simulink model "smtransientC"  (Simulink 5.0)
settings: Solver=ode45  StartTime=0.0  StopTime=2  MaxStep=1e-3  RelTol=1e-4  AbsTol=1e-4
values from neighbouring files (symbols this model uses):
  Bm = 0.10    (= 0.1)    [IMabc2.m]    (also in imabcparam.m = 0.01; IMabcrun0.m = 0.01; IMabcrun1.m = 0.001; IMcur0.m = 1e-06)
  H = 0.60    (= 0.6)    [IMabc2.m]    (also in IMcur0.m = 0.3; imdef0vec.m = 0.3; imdef1vec.m = 0.3; imdef2vec.m = 0.3)
  n0 = 0.98    [imdef0vec.m]    (also in imdef1vec.m = 0.978; imdef2vec.m; imdefrotflux.m; imdefSIvec1.m = 0.95)
  tc = abs(fco)    [im3phase.m]
  Te0 = 0.75/wo*p*(Is*conj(Is)*Req)    [imdefSIvec1.m]
  V = [Vas 0 0].'    [Actac.m]    (also in acttrcalc1.m = str2num(get(h,'string')); im3d.m = eval(get(hVs,'String')); IMabc2.m = [vas vbs vcs 0 0 0]'; IMabcf0.m = [vas vbs vcs 0 0 0]')
  wo = 2*pi*freq0    [calc0.m]    (also in IMabc2.m = 376.991118431; imabcparam.m = 376.991118431; IMabcrun0.m = 376.991118431; IMabcrun1.m = 376.991118431)
undefined symbols (not defined in the file or in its folder): delta0, Lw_1, phif0
libraries: simulink x1

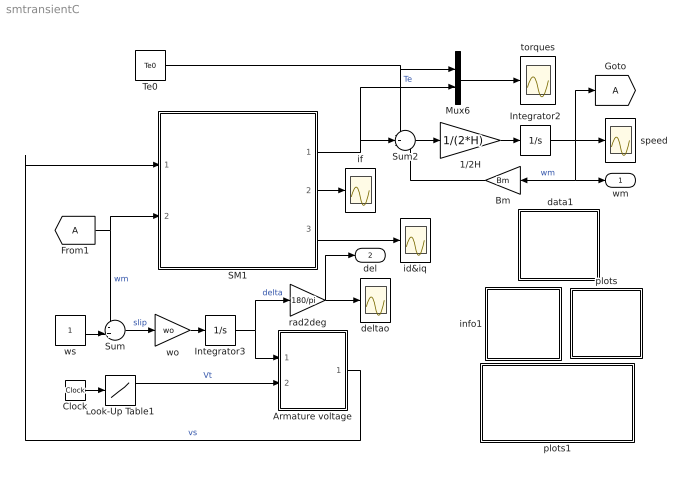
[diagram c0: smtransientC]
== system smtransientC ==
  " data1" : Subsystem
  1/2H : Gain  Gain=1/(2*H)
  Armature voltage : Subsystem
  Bm : Gain  Orientation=left  Gain=Bm
  Clock : Clock
  Integrator2 : Integrator  InitialCondition=n0
  Integrator3 : Integrator  InitialCondition=delta0
  Look-Up Table1 : Lookup  InputValues=[0 0.5 0.5 0.5+tc 0.5+tc 3]  OutputValues=[V V 0 0 V V]
  Mux6 : Mux  Inputs=2
  SM1 : Subsystem
  Sum : Sum  Inputs=-+|
  Sum2 : Sum  Inputs=-+-
  Te0 : Constant  Value=Te0
  deltao : Scope
  id&iq : Scope
  if : Scope
  info1 : Subsystem
  plots : Subsystem
  plots1 : Subsystem
  rad2deg : Gain  Gain=180/pi
  speed : Scope
  torques : Scope
  wo : Gain  Gain=wo
  ws : Constant
  wm : Outport
  del : Outport  Port=2
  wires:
  Mux6/1 -> torques/1
  SM1/2(if) -> if/1
  Sum2/1 -> 1/2H/1
  1/2H/1 -> Integrator2/1
  SM1/1(Te) -> Sum2/2, Mux6/2  "Te"
  Bm/1 -> Sum2/3
  Integrator2/1 -> speed/1, [A], Bm/1, wm/1  "wm"
  Te0/1 -> Mux6/1, Sum2/1
  ws/1 -> Sum/2
  Sum/1 -> wo/1  "slip"
  wo/1 -> Integrator3/1
  Armature voltage/1(vs) -> SM1/1(vs)  "vs"
  Integrator3/1 -> Armature voltage/1(delta), rad2deg/1  "delta"
  SM1/3(ia) -> id&iq/1
  rad2deg/1 -> deltao/1, del/1
  Clock/1 -> Look-Up Table1/1
  Look-Up Table1/1 -> Armature voltage/2(Vt)  "Vt"
  [A] -> SM1/2(wm), Sum/1  "wm"

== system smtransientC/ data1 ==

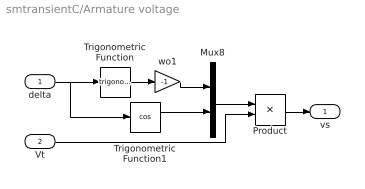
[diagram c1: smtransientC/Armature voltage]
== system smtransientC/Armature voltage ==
  delta : Inport
  Vt : Inport  Port=2
  Mux8 : Mux  Inputs=2
  Product : Product
  Trigonometric Function : Trigonometry
  Trigonometric Function1 : Trigonometry  Operator=cos
  wo1 : Gain  Gain=-1
  vs : Outport
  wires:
  delta/1 -> Trigonometric Function/1, Trigonometric Function1/1
  Trigonometric Function/1 -> wo1/1
  Mux8/1 -> Product/1
  wo1/1 -> Mux8/1
  Trigonometric Function1/1 -> Mux8/2
  Product/1 -> vs/1
  Vt/1 -> Product/2

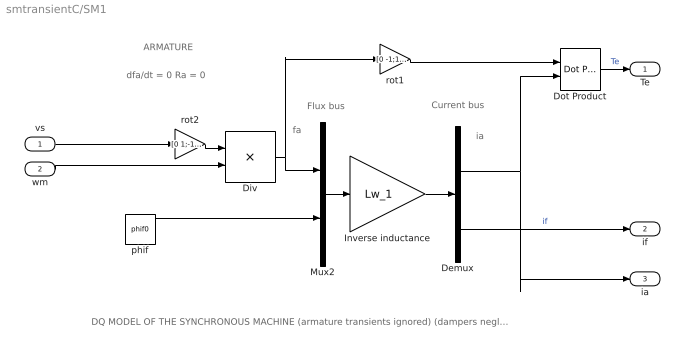
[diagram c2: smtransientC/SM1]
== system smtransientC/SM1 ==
  note: ARMATURE
  note: fa
  note: ia
  note: Flux bus
  note: Current bus
  note: dfa/dt = 0 Ra = 0
  note: DQ MODEL OF THE SYNCHRONOUS MACHINE (armature transients ignored) (dampers neglected) (constant field flux linkage)
  vs : Inport
  wm : Inport  Port=2
  Demux : Demux  Outputs=2
  Div : Product  Inputs=*/  Multiplication=Matrix(*)
  Dot Product : simulink/Math Operations/Dot Product
  Inverse inductance : Gain  Gain=Lw_1  Multiplication=Matrix(K*u)
  Mux2 : Mux  Inputs=2
  phif : Constant  Value=phif0
  rot1 : Gain  Gain=[0 -1;1 0]  Multiplication=Matrix(K*u)
  rot2 : Gain  Gain=[0 1;-1 0]  Multiplication=Matrix(K*u)
  Te : Outport
  if : Outport  Port=2
  ia : Outport  Port=3
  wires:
  rot1/1 -> Dot Product/1
  Demux/1 -> Dot Product/2, ia/1
  Dot Product/1 -> Te/1  "Te"
  Mux2/1 -> Inverse inductance/1
  Inverse inductance/1 -> Demux/1
  Demux/2 -> if/1  "if"
  vs/1 -> rot2/1
  Div/1 -> Mux2/1, rot1/1
  rot2/1 -> Div/1
  wm/1 -> Div/2
  phif/1 -> Mux2/2

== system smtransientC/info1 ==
  note: Synchronous machine transient stability
  note: This demonstration illustrates the dynamics of a synchronous machine following the sudden application and removal of a three-phase short circuit at the terminals. Four models of the synchronous machine are provided: 1) A complete model (5th-order) 2) Armature transients ignored by setting dfa/dt=0 (3rd-order) 3) Both armature transients and damper effects are neglected (1st-order) 4) Constant field flux linkage (zero-order) Click the DATA block to enter the parameters and prefault operating conditions. Initialize and then Start the simulation.

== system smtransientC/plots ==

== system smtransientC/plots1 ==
